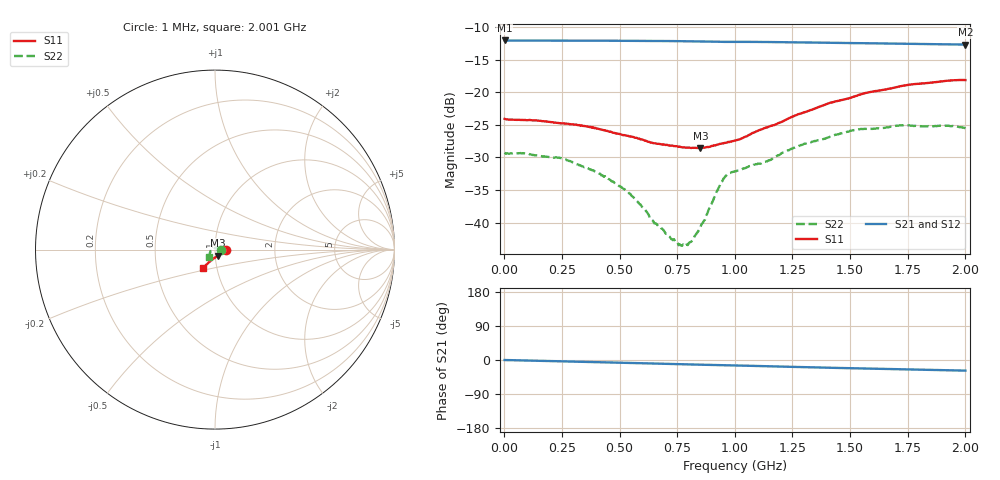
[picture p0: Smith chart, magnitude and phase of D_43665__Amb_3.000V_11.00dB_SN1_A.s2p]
! device id: 43665_
! dir: \\malibu\benchdata\1_engineers\tn_data\43665_75ohm\new\sparar\43665_\amb\3p000v\11p00db
! Serial: 1
! Insertion: A
! Temp: Amb
! VDD: 3.000V
! Attenuation Step: 11.00dB
! IDD: 1.450772e+00mA
! FILE NAME
! DATE 03-27-2009 08:36:04
! CORRECTED  DATA
#  Hz  S  RI  R  75
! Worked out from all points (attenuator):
!   401 points, 1 MHz to 2.001 GHz, reference 75 ohm
!   highest |S21| = -12.03 dB at 1 MHz (marker M1); lowest = -12.7 dB at 2.001 GHz (marker M2)
!   lowest |S11| = -28.6 dB at 851 MHz (marker M3), VSWR 1.08, Z = 77.5 - j5.11 ohm
!   |S11| at or under -10 dB: start of sweep to end of sweep
!   |S22| runs from -43.6 to -25.0 dB; largest |S21 - S12| = 0.0013
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1000000  0.0626 -0.00053  0.2502 -0.00035  0.2503 -0.000414  0.0345 -0.000354
2.36e8  0.0578 -0.00633  0.2492 -0.0145  0.2493 -0.0145  0.0302 0.00884
3.36e8  0.0549 -0.00961  0.2485 -0.0207  0.2485 -0.0207  0.0246 0.0113
4.06e8  0.0514 -0.0115  0.2479 -0.0249  0.2479 -0.0249  0.0207 0.0123
5.31e8  0.0433 -0.0169  0.2464 -0.0329  0.2464 -0.0329  0.0132 0.0115
5.91e8  0.0389 -0.0194  0.2454 -0.0365  0.2454 -0.0365  0.00773 0.0114
6.71e8  0.0328 -0.0234  0.2443 -0.0414  0.2443 -0.0414  0.00336 0.00859
7.21e8  0.0289 -0.0262  0.2434 -0.0446  0.2435 -0.0445  3.37e-05 0.00764
7.76e8  0.0245 -0.0288  0.2423 -0.0481  0.2424 -0.0481  -0.00422 0.00532
8.06e8  0.0219 -0.0304  0.2418 -0.0501  0.2417 -0.05  -0.00651 0.00276
8.51e8  0.0175 -0.0329  0.2406 -0.053  0.2406 -0.0529  -0.00925 -0.000397
9.46e8  0.00826 -0.0396  0.2371 -0.0583  0.2372 -0.0581  -0.0194 -0.00745
9.71e8  0.006 -0.0412  0.2366 -0.0591  0.2367 -0.0589  -0.0229 -0.00642
1.001e9  0.00299 -0.0424  0.2363 -0.0605  0.2365 -0.0603  -0.024 -0.00588
1.146e9  -0.0115 -0.0531  0.2332 -0.0693  0.2334 -0.0691  -0.0263 -0.0145
1.246e9  -0.0219 -0.0607  0.2303 -0.075  0.2306 -0.075  -0.0296 -0.0219
1.336e9  -0.0298 -0.0674  0.2276 -0.0797  0.228 -0.0796  -0.0319 -0.027
1.521e9  -0.0459 -0.081  0.2215 -0.0891  0.2219 -0.0893  -0.0348 -0.0378
1.671e9  -0.0557 -0.0911  0.2165 -0.0962  0.2166 -0.0965  -0.0345 -0.0417
1.741e9  -0.0598 -0.0962  0.214 -0.0993  0.2143 -0.0998  -0.0338 -0.0447
1.921e9  -0.0664 -0.1032  0.208 -0.1065  0.2081 -0.1067  -0.033 -0.0445
2.001e9  -0.0672 -0.1045  0.2054 -0.1094  0.2046 -0.1104  -0.031 -0.043
